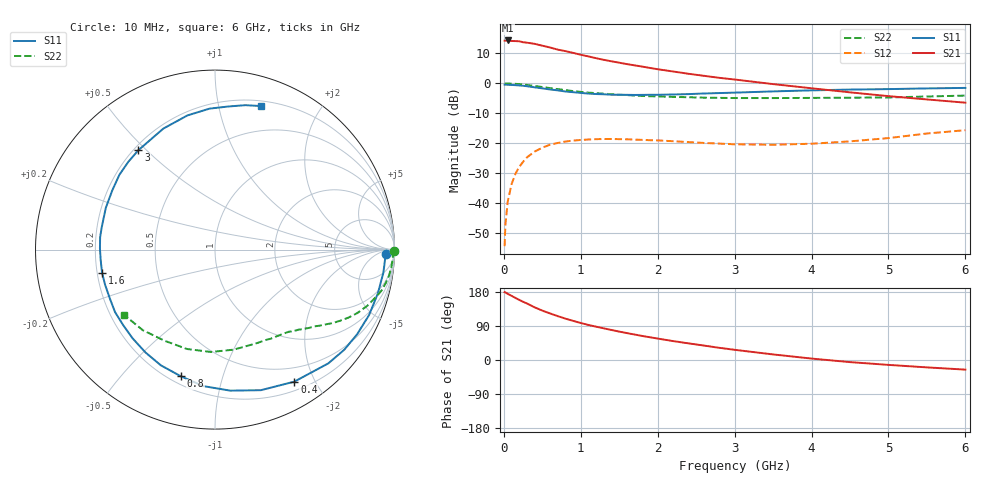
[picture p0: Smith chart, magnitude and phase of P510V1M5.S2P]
! SIEMENS Small Signal Semiconductors
! BFP183
! Si NPN RF Bipolar Junction Transistor in SOT143
! VCE = 10 V  IC = 1.5 mA
! Common Emitter S-Parameters:  March  1996
# GHz  S  MA  R  50
!  f  S11  S21  S12  S22
! GHz  MAG  ANG  MAG  ANG  MAG  ANG  MAG  ANG
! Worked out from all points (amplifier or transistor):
!   36 points, 10 MHz to 6 GHz, reference 50 ohm
!   highest |S21| = 14.3 dB at 50 MHz (marker M1)
!   |S21| within 3 dB of that: start of sweep to 691.8 MHz
!   unconditionally stable (mu >= 1): 2.346 GHz to end of sweep
!   at 250 MHz: K = 0.11, MSG = 20.0 dB, |S12| = -26.2 dB
!   at 1.4 GHz: K = 0.59, MSG = 13.0 dB, |S12| = -18.6 dB
!   at 6 GHz: K = 1.01, MAG = 3.9 dB, |S12| = -15.7 dB
!   S11 on the Smith chart (normalised r, x): 10 MHz: 33, -18; 400 MHz: 0.31, -1.73; 800 MHz: 0.24, -0.74; 1.6 GHz: 0.22, -0.10; 3 GHz: 0.22, +0.47; 6 GHz: 0.25, +1.34
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0.01  0.9544 -1.5  5.161 179.1  0.0019 85.3  0.9986 -0.5
0.02  0.9491 -3.2  5.16 178.4  0.0043 90.0  0.9887 -1.1
0.05  0.9469 -7.8  5.206 174.6  0.0105 86.8  0.9929 -2.8
0.1  0.9396 -15.0  5.107 169.4  0.0206 79.9  0.9872 -5.6
0.2  0.9217 -30.8  5.045 158.6  0.0401 72.0  0.9695 -11.1
0.4  0.8582 -59.0  4.571 139.0  0.0723 56.2  0.905 -20.2
0.5  0.824 -71.9  4.257 130.4  0.0842 49.3  0.8674 -24.1
0.6  0.7905 -83.8  3.972 122.9  0.0942 43.3  0.8332 -27.1
0.7  0.7633 -94.9  3.661 115.8  0.1008 37.8  0.7999 -29.8
0.8  0.7309 -105.1  3.454 109.2  0.1065 33.4  0.7712 -32.1
1  0.6916 -124.1  3.003 97.7  0.113 25.6  0.7198 -36.1
1.1  0.6745 -133.0  2.817 92.4  0.1152 22.4  0.6996 -37.7
1.3  0.6568 -148.0  2.469 83.5  0.1173 16.5  0.6708 -40.9
1.6  0.6424 -168.4  2.096 71.0  0.1161 10.7  0.6367 -45.1
1.8  0.6411 179.3  1.903 63.4  0.1135 8.2  0.615 -48.1
2.2  0.6513 159.1  1.578 49.9  0.1078 4.6  0.5934 -54.3
2.6  0.6765 141.9  1.336 38.1  0.1009 4.1  0.5764 -61.2
3  0.6993 127.6  1.158 26.9  0.0957 5.8  0.5675 -69.0
3.5  0.7331 113.1  0.971 14.7  0.0941 11.0  0.567 -79.5
4.5  0.7861 92.2  0.707 -5.6  0.1072 21.8  0.5753 -105.7
5.5  0.8224 78.1  0.538 -19.5  0.1451 25.5  0.6029 -131.9
6  0.839 72.4  0.475 -25.4  0.1647 22.8  0.624 -144.5
